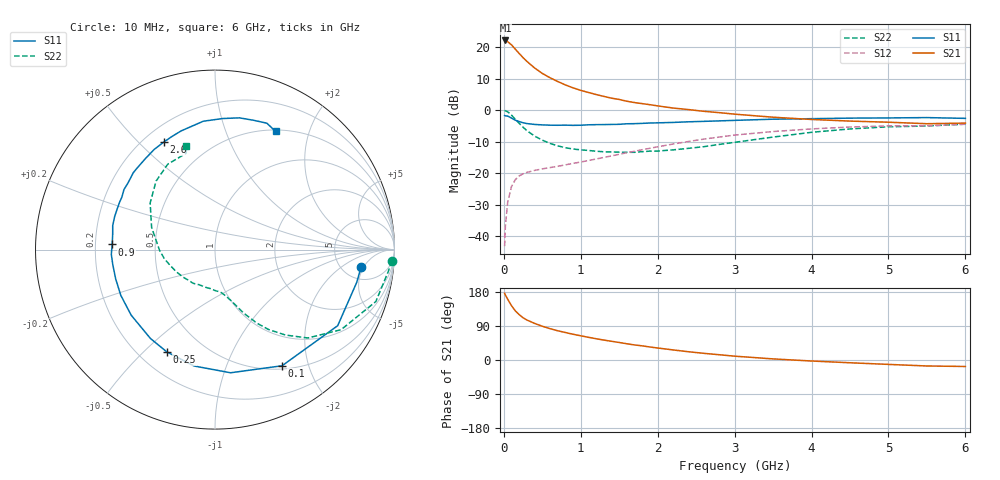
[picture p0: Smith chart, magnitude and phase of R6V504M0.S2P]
! SIEMENS Small Signal Semiconductors
! BFR193
! Si NPN RF Bipolar Junction Transistor in SOT23
! VCE = 0.5 V  IC = 4 mA
! Common Emitter S-Parameters:  May  1996
# GHz  S  MA  R  50
!  f  S11  S21  S12  S22
! GHz  MAG  ANG  MAG  ANG  MAG  ANG  MAG  ANG
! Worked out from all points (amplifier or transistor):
!   36 points, 10 MHz to 6 GHz, reference 50 ohm
!   highest |S21| = 22.1 dB at 20 MHz (marker M1)
!   |S21| within 3 dB of that: start of sweep to 158 MHz
!   unconditionally stable (mu >= 1): 891.4 MHz to 2.439 GHz; 5.287 GHz to end of sweep
!   at 250 MHz: K = 0.38, MSG = 18.4 dB, |S12| = -20.2 dB
!   at 1.4 GHz: K = 1.11, MAG = 7.1 dB, |S12| = -14.5 dB
!   at 6 GHz: K = 1.01, MAG = -0.4 dB, |S12| = -4.5 dB
!   S11 on the Smith chart (normalised r, x): 10 MHz: 7.52, -4.39; 100 MHz: 0.54, -1.60; 250 MHz: 0.31, -0.59; 900 MHz: 0.27, +0.02; 2.6 GHz: 0.28, +0.60; 6 GHz: 0.52, +1.51
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0.01  0.8201 -6.7  12.66 176.2  0.007 86.4  0.988 -3.6
0.02  0.8105 -13.0  12.68 171.7  0.0145 84.2  0.9727 -7.3
0.05  0.8044 -31.8  12.11 160.3  0.0348 73.5  0.9417 -17.9
0.1  0.7473 -60.0  10.8 143.3  0.0618 61.1  0.8324 -32.4
0.15  0.6917 -82.8  9.207 129.4  0.0794 51.3  0.7141 -43.6
0.2  0.6589 -100.2  7.869 119.7  0.0908 45.6  0.6169 -50.5
0.25  0.63 -115.2  6.777 111.5  0.098 41.4  0.5354 -56.2
0.3  0.612 -126.0  5.904 105.5  0.1031 39.3  0.4723 -60.3
0.4  0.5929 -142.0  4.651 96.5  0.1109 37.1  0.3881 -65.7
0.5  0.5834 -154.1  3.81 89.1  0.1173 36.6  0.3344 -69.3
0.6  0.577 -163.5  3.257 82.7  0.1228 37.4  0.2971 -72.7
0.7  0.5756 -171.5  2.841 77.2  0.1289 38.8  0.2718 -76.0
0.9  0.5734 177.1  2.251 68.0  0.1434 41.3  0.242 -81.8
1.1  0.5854 166.8  1.903 59.9  0.1591 43.8  0.2297 -88.9
1.3  0.5898 158.0  1.648 52.6  0.1781 45.9  0.2187 -96.8
1.6  0.6077 146.6  1.381 42.8  0.2115 47.7  0.2146 -110.3
2.2  0.6381 127.5  1.078 26.6  0.2906 45.6  0.2346 -139.1
2.6  0.6636 115.5  0.957 17.6  0.3473 41.3  0.2634 -159.9
3.5  0.7182 95.2  0.772 2.9  0.4579 27.4  0.3742 160.7
4.5  0.7465 79.5  0.67 -7.3  0.5398 11.7  0.5034 130.7
5.5  0.7612 67.7  0.609 -15.8  0.5656 -3.0  0.5601 106.6
6  0.7399 62.8  0.623 -17.1  0.5968 -7.3  0.5995 105.5
